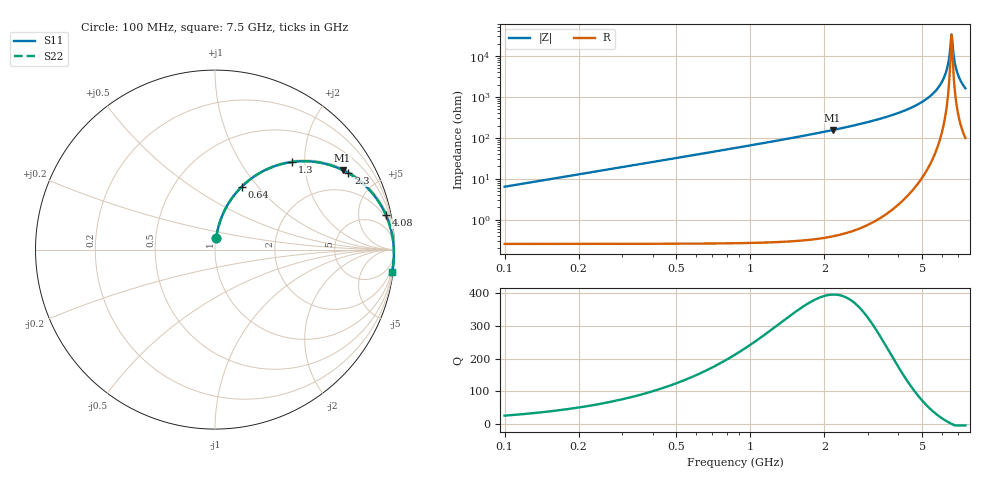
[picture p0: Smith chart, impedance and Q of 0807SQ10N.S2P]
! Coilcraft 0807SQ-10N Air Core Inductor
! 06 March 2008
# MHZ S MA R 50
!Freq  MagS11  AngS11  MagS21  AngS21  MagS12  AngS12  MagS22  AngS22
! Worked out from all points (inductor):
!   371 points, 100 MHz to 7.5 GHz, reference 50 ohm
!   read as one part in series: L = 10.2 nH near 120 MHz
!   highest Q = 396 at 2.16 GHz (marker M1), where L = 11.4 nH
!   self-resonance near 6.58 GHz
!   S11 on the Smith chart (normalised r, x): 100 MHz: 1.01, +0.13; 640 MHz: 1.01, +0.82; 1.3 GHz: 1.02, +1.74; 2.3 GHz: 1.07, +3.44; 4.08 GHz: 1.42, +9.82; 7.5 GHz: 1, -16
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100  0.06336 84.0  0.9954 -3.7  0.9954 -3.7  0.06337 84.0
180  0.1135 82.1  0.991 -6.6  0.991 -6.6  0.1135 82.1
300  0.1873 78.3  0.9798 -10.9  0.9798 -10.9  0.1873 78.3
640  0.3792 67.1  0.9229 -22.6  0.9229 -22.6  0.3792 67.1
1300  0.6512 48.6  0.7567 -41.2  0.7567 -41.2  0.6512 48.6
1340  0.6634 47.6  0.7461 -42.2  0.7461 -42.2  0.6635 47.6
2160  0.8378 31.9  0.5438 -57.9  0.5438 -57.9  0.8379 31.9
2300  0.8567 29.8  0.5136 -60.0  0.5136 -60.0  0.8567 29.8
2580  0.888 26.0  0.4575 -63.8  0.4575 -63.8  0.888 26.0
3800  0.9629 13.6  0.2649 -76.1  0.2649 -76.1  0.963 13.6
4080  0.9718 11.4  0.2299 -78.3  0.2299 -78.3  0.9718 11.4
5040  0.99 4.9  0.1273 -84.2  0.1273 -84.2  0.99 4.9
5820  0.9959 0.6  0.05859 -87.1  0.05859 -87.1  0.996 0.6
6080  0.9967 -0.7  0.03792 -86.9  0.03792 -86.9  0.9968 -0.7
6280  0.997 -1.7  0.0227 -84.9  0.0227 -84.9  0.9971 -1.7
6440  0.9971 -2.5  0.01104 -77.7  0.01104 -77.7  0.9972 -2.5
6580  0.997 -3.1  0.002966 -13.7  0.002966 -13.7  0.9971 -3.1
6600  0.997 -3.2  0.003061 13.6  0.003061 13.6  0.9971 -3.2
6720  0.9969 -3.7  0.009835 68.3  0.009835 68.3  0.997 -3.7
6880  0.9966 -4.5  0.02065 76.7  0.02065 76.7  0.9967 -4.5
7140  0.9959 -5.6  0.03796 79.3  0.03796 79.3  0.9959 -5.6
7500  0.9944 -7.1  0.06095 79.4  0.06095 79.4  0.9945 -7.1
